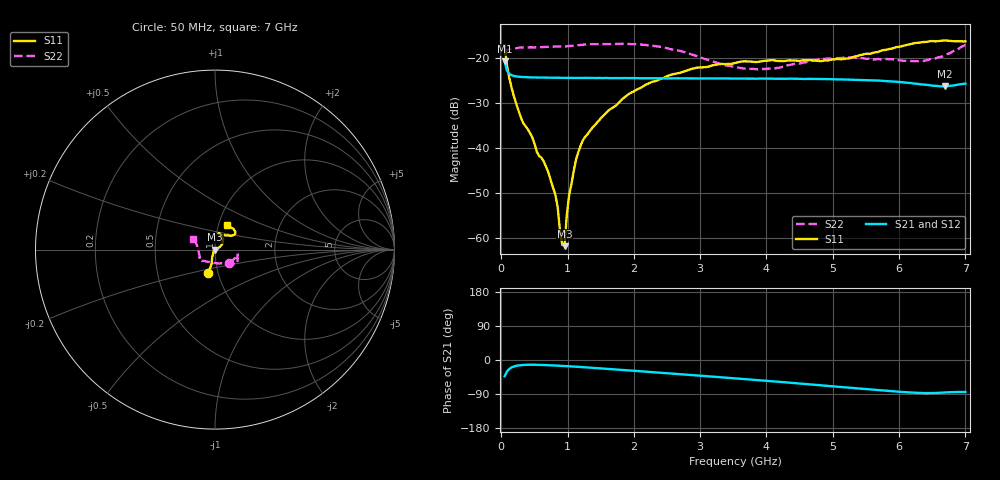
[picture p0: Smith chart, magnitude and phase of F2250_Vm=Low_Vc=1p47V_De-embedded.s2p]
! Integrated Device Technology
! Corporate Headquarters
! 6024 Silver Creek Valley Road
! San Jose, CA 95138  USA
! Phone:  1-408-284-8200
! Toll Free:  1-800-223-1366
! Webpage:  http://www.idt.com/
! Timing and RF Division
! 515 Groton Road, Suite 102
! Westford, MA 01886-6024
! Device:  F2250
! Description: Voltage Variable RF Attenuator
! Frequency:  50.0 -  6000.00 MHz
! Package:  3x3 mm Thin QFN Plastic Package: 16 pin
! Ports:  2 RF, 3 DC
!  Pin  1  = GND
!  Pin  2  = NC
!  Pin  3  = RF1  = Port 1
!  Pin  4  = NC
!  Pin  5  = GND
!  Pin  6  = GND
!  Pin  7  = GND
!  Pin  8  = GND
!  Pin  9  = NC
!  Pin 10  = RF2  = Port 2
!  Pin 11  = NC
!  Pin 12  = GND
!  Pin 13  = GND
!  Pin 14  = VCNTRL
!  Pin 15  = VDD
!  Pin 16  = VMODE
! Vcntrl:  1.470 Volts
! Vmode:  +0.000 Volts
! Vdd:  +3.30  Volts
! Current:  1.191 mA
! Data:  The device was measured on a the F2250 evaluation board which has
!  individual transmission lines to the RF pins.  Data was collected
!  using a calibrated network analyzer.  The evaluation board was
!  de-embedded using a TRL calibration technique.
!  The reference plane is the edge of the package pin.
! Misc:  SN 10
!  Action Tracker AT0258
! Date Measured:  2014-11-26
! Date:  2015-10-15  MJV
! Note:
!  Integrated Device Technology supplies this data as a sample of measured
!  data at the package pin for this product.  Your particular data for this
!  product may vary.
!  Data was taken at 25 degrees C.
!  Integrated Device Technology reserves the right to change this data at anytime.
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# GHz S dB R 50
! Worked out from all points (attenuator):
!   201 points, 50 MHz to 7 GHz, reference 50 ohm
!   highest |S21| = -20.86 dB at 50 MHz (marker M1); lowest = -26.4 dB at 6.687 GHz (marker M2)
!   lowest |S11| = -61.7 dB at 953.5 MHz (marker M3), VSWR 1.00, Z = 50 - j0.0812 ohm
!   |S11| at or under -10 dB: start of sweep to end of sweep
!   |S22| runs from -22.6 to -16.9 dB; largest |S21 - S12| = 0.00025
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0.05  -17.27 -105.8  -20.86 -42.9  -20.86 -42.9  -19.06 -43.9
0.1195  -24.45 -106.2  -23.57 -23.7  -23.60 -23.7  -18.19 -16.0
0.29325  -33.17 -114.4  -24.28 -13.6  -24.27 -13.6  -17.75 -11.8
0.64075  -43.00 -135.2  -24.44 -13.3  -24.42 -13.2  -17.66 -15.3
0.8145  -50.27 -171.3  -24.48 -14.6  -24.47 -14.6  -17.58 -18.8
0.84925  -53.01 -172.7  -24.49 -14.9  -24.48 -14.9  -17.53 -19.6
0.884  -58.11 177.4  -24.48 -15.2  -24.47 -15.2  -17.52 -20.3
0.91875  -61.41 128.2  -24.50 -15.6  -24.49 -15.5  -17.50 -21.1
0.9535  -61.73 -98.0  -24.52 -15.9  -24.49 -15.9  -17.58 -21.5
0.98825  -54.77 -17.5  -24.49 -16.2  -24.48 -16.2  -17.50 -21.9
1.023  -50.44 -3.5  -24.48 -16.6  -24.48 -16.6  -17.45 -22.1
1.12725  -42.56 13.8  -24.49 -17.7  -24.47 -17.7  -17.30 -23.9
1.2315  -38.26 17.9  -24.50 -18.9  -24.49 -18.8  -17.13 -25.8
1.857  -28.80 31.7  -24.52 -26.6  -24.53 -26.6  -16.93 -32.4
2.37825  -24.85 41.6  -24.58 -33.3  -24.57 -33.3  -17.57 -37.6
3.525  -21.20 69.9  -24.64 -48.5  -24.63 -48.5  -22.09 -78.2
4.081  -20.57 77.4  -24.65 -56.1  -24.68 -56.1  -22.46 -113.2
4.7065  -20.64 71.0  -24.72 -65.1  -24.72 -65.1  -20.67 -137.1
5.85325  -18.09 39.0  -25.25 -81.8  -25.23 -81.9  -20.39 -154.0
6.33975  -16.62 40.0  -25.94 -87.0  -25.94 -87.1  -20.80 -172.9
6.68725  -16.21 48.0  -26.38 -85.7  -26.36 -85.7  -19.43 164.2
7  -16.41 62.8  -25.75 -84.4  -25.74 -84.4  -17.20 154.8
